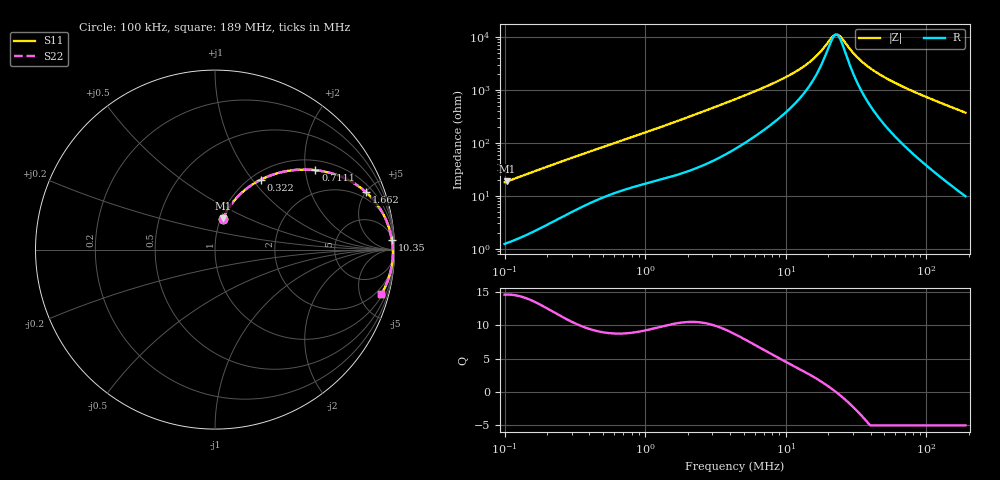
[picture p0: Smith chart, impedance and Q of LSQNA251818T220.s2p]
! LSQNA251818T220  S-PARAMETER MODEL  ( General Type )
! Model Generated by TAIYO YUDEN Corporation (http://www.ty-top.com)
! Version 2.0
! TAIYO YUDEN Control No. 100810NF25SB-FKC
! Copyright(c) 2007 TAIYO YUDEN CO.,LTD. All Rights Reserved.
! Product Description (link to TY-COMPAS)
! https://ds.yuden.co.jp/TYCOMPAS/or/detail?pn=LSQNA251818T220K&u=M
! Products Name : Inductors
! Characteristics :
!  Inductance : 22 uH , SRF(min) : 19 MHz , DC Resistance(max) : 0.65 Ohm
!  Rated Current : Saturation :165 mA , Temp Rise : 580 mA (40 degC)
!  Case Size : 2.5 x 1.8 / 0.098 x 0.071 [mm/inch] , Thickness : 1.8 / 0.071 [mm/inch]
!  (Conditions: Temperature = 25 degC , DC Bias Current/Voltage = 0A / 0V)
! External Node Assignments :
!  1  o---GGG---o  2
! GND o---------o GND
! Frequency Range : 0.1MHz  -  189.042664MHz  [ 402 STEP ]
# MHz S RI R 50
! Freq[MHz].  S11 Real  S11 Imag  S21 Real  S21 Imag  S12 Real  S12 Imag  S22 Real  S22 Imag
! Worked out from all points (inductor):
!   401 points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, 100 kHz to 189 MHz, reference 50 ohm
!   read as one part in series: L = 28.3 uH near 103.8 kHz
!   highest Q = 14.6 at 103.8 kHz (marker M1), where L = 28.4 uH
!   self-resonance near 22.44 MHz
!   S11 on the Smith chart (normalised r, x): 100 kHz: 1.02, +0.36; 322 kHz: 1.11, +1.10; 711.1 kHz: 1.26, +2.27; 1.662 MHz: 1.49, +5.03; 10.35 MHz: 9, +36; 189 MHz: 1.20, -7.43
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0.1  0.042 0.1691  0.958 -0.1691  0.958 -0.1691  0.042 0.1691
0.103844  0.0446 0.1749  0.9554 -0.1749  0.9554 -0.1749  0.0446 0.1749
0.189892  0.1189 0.287  0.8811 -0.287  0.8811 -0.287  0.1189 0.287
0.322008  0.255 0.3896  0.745 -0.3896  0.745 -0.3896  0.255 0.3896
0.353854  0.2868 0.4043  0.7132 -0.4043  0.7132 -0.4043  0.2868 0.4043
0.711059  0.5593 0.4427  0.4407 -0.4427  0.4407 -0.4427  0.5593 0.4427
1.252125  0.7657 0.3752  0.2343 -0.3752  0.2343 -0.3752  0.7657 0.3752
1.66157  0.842 0.3193  0.158 -0.3193  0.158 -0.3193  0.842 0.3193
2.564016  0.9181 0.2303  0.0819 -0.2303  0.0819 -0.2303  0.9181 0.2303
4.347904  0.9622 0.1416  0.0378 -0.1416  0.0378 -0.1416  0.9622 0.1416
10.35343  0.9852 0.0519  0.0148 -0.0519  0.0148 -0.0519  0.9852 0.0519
15.38522  0.989 0.0245  0.011 -0.0245  0.011 -0.0245  0.989 0.0245
17.55672  0.9899 0.0161  0.0101 -0.0161  0.0101 -0.0161  0.9899 0.0161
21.20106  0.9908 0.00437  0.00916 -0.00437  0.00916 -0.00437  0.9908 0.00437
23.29778  0.9912 -0.00152  0.00883 0.00152  0.00883 0.00152  0.9912 -0.00152
24.65407  0.9913 -0.00508  0.00868 0.00508  0.00868 0.00508  0.9913 -0.00508
30.3385  0.9916 -0.0185  0.00844 0.0185  0.00844 0.0185  0.9916 -0.0185
35.27973  0.9914 -0.0289  0.00861 0.0289  0.00861 0.0289  0.9914 -0.0289
42.60291  0.9907 -0.0428  0.0093 0.0428  0.0093 0.0428  0.9907 -0.0428
54.44117  0.9888 -0.0633  0.0112 0.0633  0.0112 0.0633  0.9888 -0.0633
94.07583  0.9774 -0.1239  0.0226 0.1239  0.0226 0.1239  0.9774 -0.1239
189.0427  0.9268 -0.2476  0.0732 0.2476  0.0732 0.2476  0.9268 -0.2476
